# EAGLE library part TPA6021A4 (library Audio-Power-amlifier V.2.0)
The TPA6021A4 is a Texas Instruments stereo audio power amplifier that drives 2 W/channel of continuous RMS power into a 4-W load when utilizing a heat sink. Advanced dc volume control minimizes external components and allows BTL (speaker) volume control and SE (headphone) volume control.
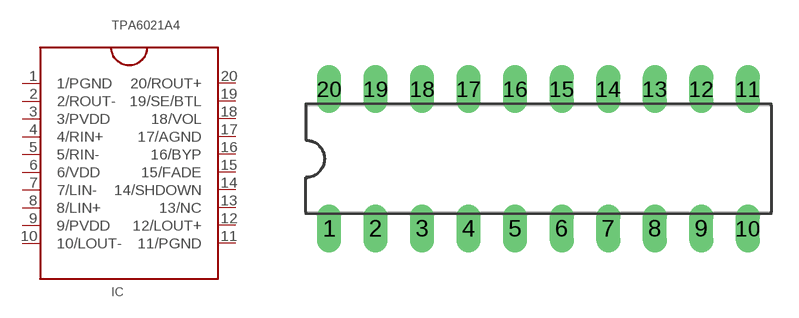
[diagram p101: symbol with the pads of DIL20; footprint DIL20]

Designator prefix IC

## TPA6021A4  [DIL20]
1  1/PGND  pwr
2  2/ROUT-  out
3  3/PVDD  pwr
4  4/RIN+  in
5  5/RIN-  in
6  6/VDD  pwr
7  7/LIN-  in
8  8/LIN+  in
9  9/PVDD  pwr
10  10/LOUT-  out
11  11/PGND  pwr
12  12/LOUT+  out
13  13/NC  nc
14  14/SHDOWN
15  15/FADE
16  16/BYP
17  17/AGND  pwr
18  18/VOL  in
19  19/SE/BTL
20  20/ROUT+  out

## Footprint DIL20 (pad centres in mm)
Dual In Line Package
drill 0.813 long: 1 -11.43,-3.81; 2 -8.89,-3.81; 3 -6.35,-3.81; 4 -3.81,-3.81; 5 -1.27,-3.81; 6 1.27,-3.81; 7 3.81,-3.81; 8 6.35,-3.81; 9 8.89,-3.81; 10 11.43,-3.81; 11 11.43,3.81; 12 8.89,3.81; 13 6.35,3.81; 14 3.81,3.81; 15 1.27,3.81; 16 -1.27,3.81; 17 -3.81,3.81; 18 -6.35,3.81; 19 -8.89,3.81; 20 -11.43,3.81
